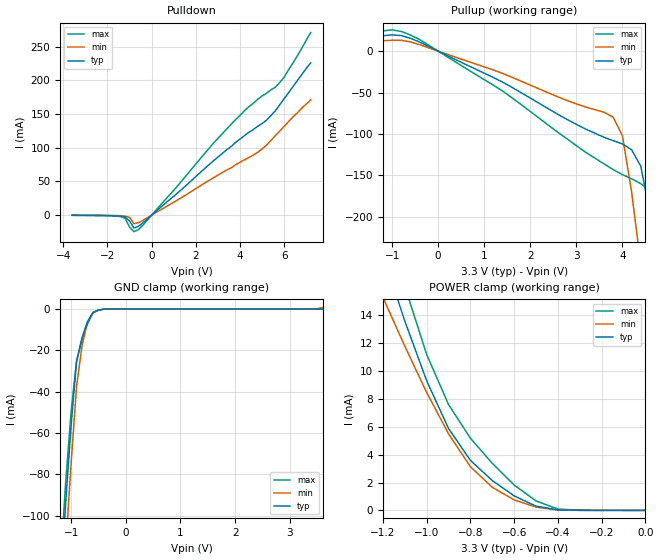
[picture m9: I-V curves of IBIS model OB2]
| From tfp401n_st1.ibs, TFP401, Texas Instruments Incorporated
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|   OUTPUT  MODEL
[Model]   OB2
Model_type   3-state
| Signals   ODCK
| variable   typ   min   max
C_comp   2pF   NA   NA
|   typ   min   max
[Temperature Range] 25.0   70.0   0.0
[Voltage range]   3.3V   3.0V   3.6V
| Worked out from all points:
|   slope of the pulldown table from 0 to 0.495 V, typ, clamps not added: 35.2 ohm
|   slope of the pullup table from 0 to 0.495 V, typ, clamps not added: 37.2 ohm
|   GND clamp passes 1 mA (typ) near -0.55 V on its own axis
|   POWER clamp passes 1 mA (typ) near -0.59 V on its own axis
[GND_clamp]
|Voltage   I(typ)   I(min)   I(max)
-3.6V     -1.31A     -1.33A     -1.29A
-1.2V     -137mA     -160mA     -126mA
-1.1V     -94.2mA    -116mA     -84.1mA
-1V       -56.4mA    -74.9mA    -49.8mA
-900mV    -25.3mA    -37.4mA    -25.1mA
-800mV    -13.8mA    -17.8mA    -14.8mA
-700mV    -6.06mA    -6.3mA     -7.18mA
-600mV    -1.6mA     -1.77mA    -1.85mA
-500mV    -470uA     -550uA     -533uA
-400mV    -39.6uA    -67.8uA    -38.2uA
3.3V      413pA      2.96uA     317pA
3.6V      1.46uA     748uA      402pA
[Power_clamp]
|Note that the [Power_clamp] voltage table is referenced to Vcc
|and is calculated using Vtable=Vcc-Vmeasured.
|Voltage   I(typ)   I(min)   I(max)
-3.3V     133mA      96.1mA     168mA
-1.2V     18.4mA     15.3mA     21.7mA
-1.1V     13.6mA     11.8mA     16.1mA
-1V       9.31mA     8.47mA     11.2mA
-900mV    5.88mA     5.5mA      7.6mA
-800mV    3.59mA     3.13mA     5.18mA
-700mV    2.14mA     1.66mA     3.38mA
-600mV    1.04mA     752uA      1.82mA
-500mV    302uA      233uA      676uA
-400mV    35.9uA     29uA       94uA
-300mV    2.26uA     2.87uA     7.04uA
0V        235pA      318pA      252pA
[Pulldown]
|Voltage   I(typ)   I(min)   I(max)
-3.6V     -246uA     -169uA     -320uA
-1.4V     -1.4mA     -788uA     -2.11mA
-1.2V     -2.91mA    -1.55mA    -4.83mA
-1V       -8.77mA    -3.29mA    -17.8mA
-800mV    -19.1mA    -12.8mA    -24.5mA
-600mV    -16.6mA    -11.3mA    -21.6mA
3.8V      108mA      74.8mA     142mA
4.6V      127mA      89.1mA     166mA
5.2V      141mA      104mA      181mA
5.6V      155mA      118mA      190mA
6V        173mA      132mA      205mA
7.2V      226mA      171mA      271mA
[Pullup]
|Note that the [Pullup] voltage table is referenced to Vcc
|and is calculated using Vtable=Vcc-Vmeasured.
|Voltage   I(typ)   I(min)   I(max)
-3.2V     5.46mA     4.2mA      6.88mA
-800mV    18.8mA     13.1mA     23.7mA
1.4V      -37.5mA    -26.9mA    -48.2mA
3.6V      -104mA     -73.7mA    -136mA
3.8V      -108mA     -79.7mA    -143mA
4V        -112mA     -102mA     -149mA
4.2V      -119mA     -170mA     -154mA
4.4V      -139mA     -258mA     -160mA
4.6V      -197mA     -351mA     -168mA
4.8V      -284mA     -446mA     -189mA
5V        -377mA     -543mA     -237mA
6.6V      -1.16A     -1.33A     -999mA
[Ramp]
|   typ   min   max
dV/dt_r   1.97v/0.71ns   1.78v/1.10ns   2.15v/0.48ns
dV/dt_f   1.97v/0.51ns   1.78v/0.81ns   2.15v/0.33ns
R_load = 5K
